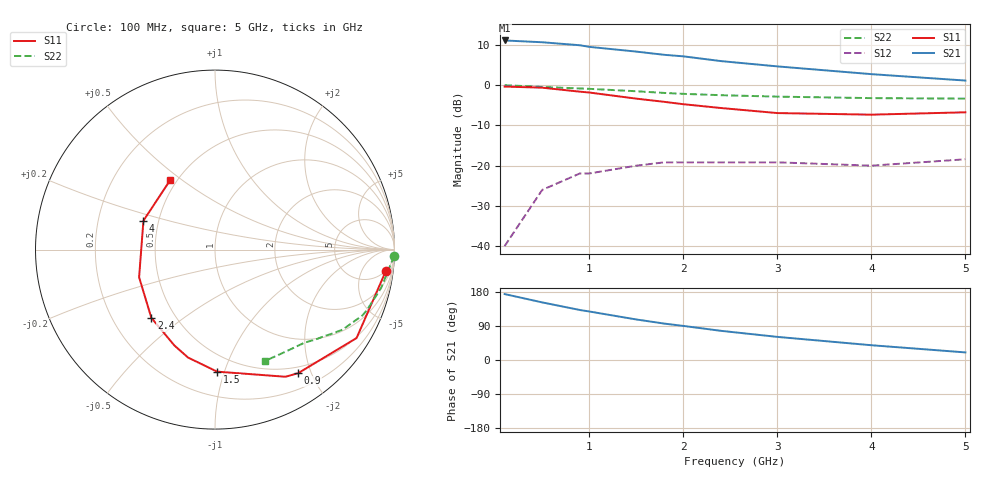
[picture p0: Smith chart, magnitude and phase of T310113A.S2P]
!AT-31011
!S and NOISE PARAMETERS at Vce=2.7V  Ic=1mA.  LAST UPDATED 06-23-94
# ghz s ma r 50
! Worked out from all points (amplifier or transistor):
!   11 points, 100 MHz to 5 GHz, reference 50 ohm
!   highest |S21| = 11.1 dB at 100 MHz (marker M1)
!   |S21| within 3 dB of that: start of sweep to 1.586 GHz
!   unconditionally stable (mu >= 1): 3.022 GHz to end of sweep
!   at 500 MHz: K = 0.19, MSG = 18.3 dB, |S12| = -26.0 dB
!   at 1.8 GHz: K = 0.55, MSG = 13.4 dB, |S12| = -19.2 dB
!   at 5 GHz: K = 1.31, MAG = 6.5 dB, |S12| = -18.4 dB
!   lowest NFmin = 0.50 dB at 500 MHz
!   S11 on the Smith chart (normalised r, x): 100 MHz: 5, -15; 900 MHz: 0.41, -1.81; 1.5 GHz: 0.37, -0.95; 2.4 GHz: 0.37, -0.38; 4 GHz: 0.41, +0.16; 5 GHz: 0.46, +0.45
0.1  0.96 -7.0  3.59 174.0  0.01 86.0  0.999 -2.0
0.5  0.93 -32.0  3.41 152.0  0.05 69.0  0.95 -13.0
0.9  0.83 -56.0  3.13 132.0  0.08 55.0  0.91 -22.0
1  0.81 -61.0  2.99 128.0  0.08 53.0  0.9 -24.0
1.5  0.68 -89.0  2.61 107.0  0.1 40.0  0.84 -32.0
1.8  0.62 -104.0  2.38 96.0  0.11 34.0  0.8 -36.0
2  0.58 -113.0  2.28 90.0  0.11 31.0  0.78 -38.0
2.4  0.52 -133.0  1.99 77.0  0.11 27.0  0.75 -42.0
3  0.45 -160.0  1.71 61.0  0.11 25.0  0.72 -46.0
4  0.43 158.0  1.37 39.0  0.1 29.0  0.69 -56.0
5  0.46 123.0  1.14 20.0  0.12 41.0  0.68 -66.0
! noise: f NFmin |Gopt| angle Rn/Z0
0.5  0.5  0.92  13  0.85
0.9  0.6  0.85  29  0.73
1.8  1.1  0.68  67  0.46
2.4  1.6  0.55  98  0.28
